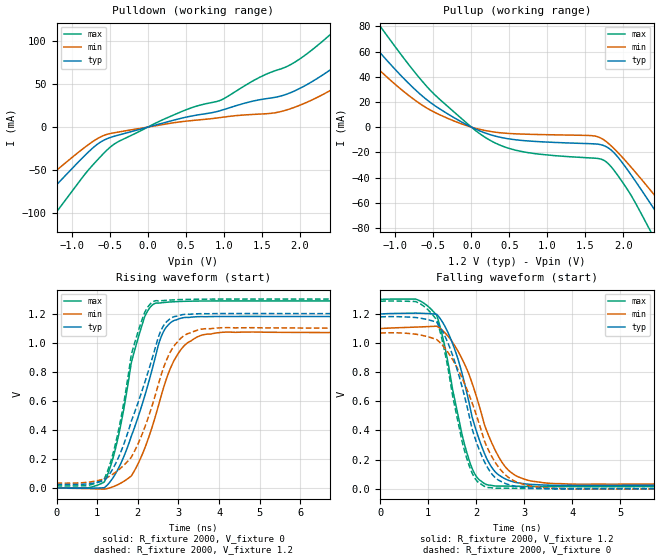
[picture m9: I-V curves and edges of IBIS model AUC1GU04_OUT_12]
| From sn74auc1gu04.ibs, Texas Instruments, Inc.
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[Model]   AUC1GU04_OUT_12
Model_type  Output
Vref =   0
Rref =   2000
Cref =   15p
Vmeas =   0.6
| variable   typ   min   max
C_comp   4.08pF   2.01pF   5.67pF
| C_pullup   3.43pF   2.01pF   4.76pF
| C_pulldown   4.72pF   4.02pF   5.67pF
[Temperature Range]   40   100   -40
| Ambient temperature   25   85   -40
[Voltage range]   1.2   1.1   1.3
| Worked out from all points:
|   slope of the pulldown table from 0 to 0.18 V, typ, clamps not added: 42.4 ohm
|   slope of the pullup table from 0 to 0.18 V, typ, clamps not added: 39 ohm
|   rising waveform, R_fixture 2000, V_fixture 0: 20-80 % time 785ps typ, 770ps min, 567ps max; typ from 0 V to 1.18 V
|   falling waveform, R_fixture 2000, V_fixture 1.2: 20-80 % time 608ps typ, 711ps min, 484ps max; typ from 1.2 V to 0.024 V
|   rising waveform, R_fixture 2000, V_fixture 1.2: 20-80 % time 831ps typ, 808ps min, 548ps max; typ from 0.024 V to 1.2 V
|   falling waveform, R_fixture 2000, V_fixture 0: 20-80 % time 624ps typ, 774ps min, 475ps max; typ from 1.18 V to 0 V
[Pulldown]
| AUC1GU04_OUT_12
|   Voltage   I(typ)   I(min)   I(max)
-3.6V     -290.8mA   -236.9mA   -365.9mA
-2.055V   -147.2mA   -115.7mA   -195.3mA
-1.775V   -121mA     -93.98mA   -164mA
-1.325V   -78.83mA   -59.6mA    -113mA
-725mV    -24.43mA   -16.91mA   -44.29mA
-450mV    -10.86mA   -6.7mA     -20.27mA
1.715V    35.36mA    17.33mA    66.67mA
2.045V    47.01mA    26.99mA    81.96mA
2.51V     73.25mA    48.06mA    116.1mA
3.08V     113.2mA    82.04mA    163.4mA
3.585V    152.5mA    117.3mA    206.9mA
7.2V      466.9mA    432.6mA    526.3mA
[Pullup]
| AUC1GU04_OUT_12
|   Voltage   I(typ)   I(min)   I(max)
-3.6V     251.1mA    225.4mA    281.8mA
-1.78V    101.5mA    81.27mA    128.7mA
-1.52V    81.86mA    64.02mA    106.8mA
-1.195V   58.57mA    44.35mA    79.56mA
-580mV    21.38mA    14.86mA    31.76mA
95mV      -2.613mA   -1.534mA   -4.567mA
640mV     -10.41mA   -5.448mA   -19.07mA
1.75V     -14.84mA   -10.39mA   -26.55mA
2.375V    -62.27mA   -51.37mA   -84.53mA
2.62V     -84.81mA   -69.62mA   -112.6mA
2.755V    -97.36mA   -79.85mA   -128mA
7.2V      -512.5mA   -430.3mA   -624.6mA
[Ramp]
| AUC1GU04_OUT_12
| variable   typ   min   max
dV/dt_r   0.71/8.52E-10   0.65/8.57E-10   0.77/6.64E-10
dV/dt_f   0.71/6.53E-10   0.65/8.12E-10   0.77/5.22E-10
R_load = 2000
[Rising Waveform]
| AUC1GU04_OUT_12
R_fixture =   2000
C_fixture =   0
L_fixture =   0
V_fixture =   0
V_fixture_min = 0
V_fixture_max = 0
|   Time   V(typ)   V(min)   V(max)
0s        3.214nV    6.297nV    2.966nV
1.18ns    1.96mV     -8.684mV   42.36mV
1.485ns   114mV      18.91mV    309.7mV
1.995ns   477.4mV    159.7mV    1.019V
2.205ns   666.2mV    298.2mV    1.199V
2.455ns   926.4mV    513.8mV    1.272V
2.69ns    1.103V     738.5mV    1.278V
3.095ns   1.171V     964.2mV    1.284V
4.11ns    1.18V      1.072V     1.288V
34.99ns   1.18V      1.069V     1.287V
[Falling Waveform]
| AUC1GU04_OUT_12
R_fixture =   2000
C_fixture =   0
L_fixture =   0
V_fixture =   1.2
V_fixture_min = 1.1
V_fixture_max = 1.3
|   Time   V(typ)   V(min)   V(max)
0s        1.2V       1.1V       1.3V
795ps     1.205V     1.111V     1.295V
1.24ns    1.172V     1.103V     1.121V
1.58ns    930.2mV    967.2mV    568.5mV
1.875ns   553.4mV    761.4mV    174.2mV
2.135ns   272.5mV    483.5mV    43.56mV
2.39ns    118.2mV    268.2mV    18.95mV
2.88ns    39.57mV    80.75mV    16.68mV
4.04ns    22.74mV    31.32mV    14.01mV
34.99ns   23.98mV    33.83mV    14.15mV
[Rising Waveform]
| AUC1GU04_OUT_12
R_fixture =   2000
C_fixture =   0
L_fixture =   0
V_fixture =   1.2
V_fixture_min = 1.1
V_fixture_max = 1.3
|   Time   V(typ)   V(min)   V(max)
0s        23.98mV    33.83mV    14.15mV
1.18ns    51.88mV    62.68mV    65.67mV
1.5ns     194.2mV    118mV      363.4mV
1.895ns   500mV      239.2mV    971.9mV
2.17ns    724.8mV    415.8mV    1.208V
2.44ns    974.1mV    647.7mV    1.289V
2.67ns    1.132V     855mV      1.291V
3.035ns   1.189V     1.024V     1.296V
4.04ns    1.2V       1.103V     1.3V
34.99ns   1.2V       1.1V       1.3V
[Falling Waveform]
| AUC1GU04_OUT_12
R_fixture =   2000
C_fixture =   0
L_fixture =   0
V_fixture =   0
V_fixture_min = 0
V_fixture_max = 0
|   Time   V(typ)   V(min)   V(max)
0s        1.18V      1.069V     1.287V
735ps     1.176V     1.061V     1.285V
1.175ns   1.143V     1.024V     1.159V
1.48ns    941.4mV    901.8mV    694.2mV
1.8ns     576.1mV    687.5mV    211.2mV
1.995ns   328.5mV    512.9mV    61.28mV
2.255ns   134.8mV    265.5mV    8.088mV
2.825ns   16.16mV    48.45mV    2.658mV
4.025ns   -954.5uV   -1.968mV   -111.9uV
34.99ns   104.3nV    226nV      33.97nV
